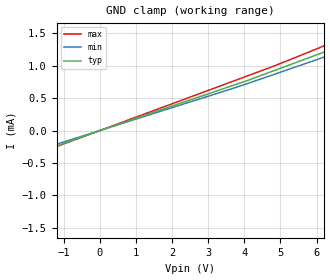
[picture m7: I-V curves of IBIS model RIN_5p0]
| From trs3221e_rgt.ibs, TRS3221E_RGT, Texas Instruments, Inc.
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[Model]   RIN_5p0
Model_type   Input
Vinl = 0.8
Vinh = 2.4
|   typ   min   max
C_comp   1.05pF   0.83pF   1.39pF
[Voltage Range]   5   4.5   5.5
[Temperature Range]   27   110   -40
[Power Clamp Reference]   5   4.5   5.5
[GND Clamp Reference]   0   0   0
[GND Clamp]
|   Voltage   I(typ)   I(min)   I(max)
-25V      -5.173mA   -4.828mA   -5.656mA
-11.64V   -2.393mA   -2.232mA   -2.618mA
-6.641V   -1.353mA   -1.262mA   -1.481mA
-3.141V   -625.6uA   -582.6uA   -685.6uA
-1.264V   -251.4uA   -222.5uA   -260.8uA
-43.29mV  -8.06uA    -7.513uA   -8.819uA
3.746V    705.9uA    660.3uA    771.1uA
4.874V    932.7uA    873.7uA    1.004mA
6.752V    1.32mA     1.236mA    1.427mA
8.416V    1.664mA    1.558mA    1.804mA
8.713V    1.725mA    1.616mA    1.871mA
25V       5.106mA    4.777mA    5.57mA
